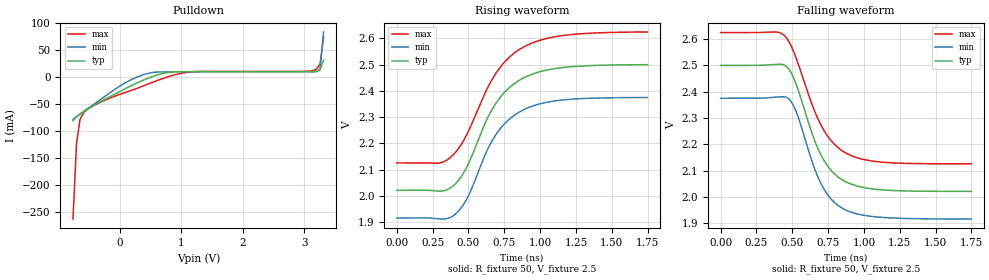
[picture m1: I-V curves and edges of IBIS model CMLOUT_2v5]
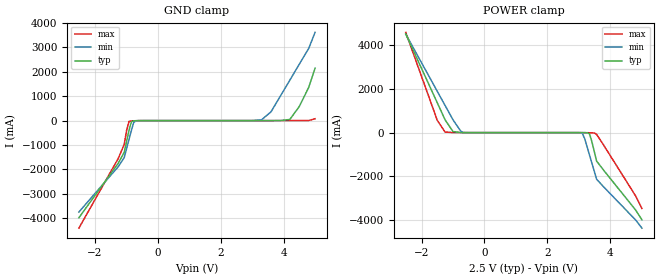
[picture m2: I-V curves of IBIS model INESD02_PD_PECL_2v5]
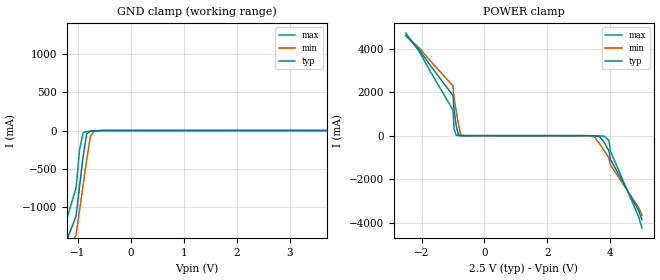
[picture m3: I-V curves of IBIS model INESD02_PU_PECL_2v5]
|   This file is an IBIS representation of the   |
|   Integrated Devices Technolog, Inc.   |
|   ICS845252I   |
|   FEMTOCLOCK CRYSTAL-TO-CML CLOCK GENERATOR   |
[IBIS Ver]   4.1
[File name]   845252i.ibs
[File Rev]   1
[Date]   9 Aug 2010
[Source]   Originated at Integrated Device Technology, Inc.
[Disclaimer]
IDT hereby grants the user of this IBIS model a non-exclusive,
nontransferable license to use this IBIS model under the following terms.
Before using this IBIS model, the user should read this license.
If the user does not accept these terms,  the IBIS model should be
returned to IDT within 30 days.
   The user is granted this license only to use the IBIS model and
is not granted rights to sell, load, rent, lease or license the IBIS
model in whole or in part, or in modified form to anyone other than
user. User may modify the IBIS model to suit its specific
applications but rights to derivative works and such modifications
shall belong to IDT.
   This IBIS model is provided on an "AS IS" basis and IDT makes
absolutely no warranty with respect to the information contained
herein. IDT DISCLAIMS AND CUSTOMER WAIVES ALL WARRANTIES, EXPRESS
OR IMPLIED, INCLUDING WARRANTIES OF MERCHANTABILITY OR FITNESS FOR
A PARTICULAR PURPOSE. The entire risk as to quality and performance
is with the Customer. ACCORDINGLY, IN NO EVENT SHALL THE COMPANY BE
LIABLE FOR ANY DAMAGES, WHETHER IN CONTRACT OR TORT,INCLUDING ANY
LOST PROFITS OR OTHER INCIDENTAL, CONSEQUENTIAL, EXEMPLARY, OR
PUNITIVE DAMAGES ARISING OUT OF THE USE OR APPLICATION OF THE IBIS
model provided in this package. Further, IDT reserves the right to
make changes without notice to any product herein to improve
reliability, function, or design. IDT does not convey any license
under patent rights or any other intellectual property rights,
including those of third parties.
   IDT is not obligated to provide maintenance or support
for the licensed IBIS model.
[Copyright]   Copyright 2010 by Integrated Device Technology, Inc.
[Component]   ICS845252KI
[Manufacturer] Integrated Device Technology, Inc.
[Package]
|LD QFN 32
|lead+wire  typ   min   max
R_pkg   72.4655m   58.886m   86.045m
L_pkg   1.47175nH   1.11650nH   1.77850n
C_pkg   0.07747pF   0.07444pF   0.08050p
[Pin]   signal_name   model_name  R_pin   L_pin   C_pin
1  nQ0   CMLOUT   86.045m   1.77850n  0.08050pF
2  Q0   CMLOUT   76.996m   1.55783n  0.07848pF
3  VDD   POWER   67.941m   1.33717n  0.07646pF
4  nOE   INESD02_PD_PECL   58.886m   1.11650n  0.07444pF
5  NC   NC   58.886m   1.11650n  0.07444pF
6  NC   NC   67.941m   1.33717n  0.07646pF
7  NC   NC   76.996m   1.55783n  0.07848pF
8  NC   NC   86.045m   1.77850n  0.08050pF
9  NC   NC   86.045m   1.77850n  0.08050pF
10 VDDA   POWER   76.996m   1.55783n  0.07848pF
11 nBYPASS  INESD02_PU_PECL   67.941m   1.33717n  0.07646pF
12 REF_CLK  INESD02_PD_PECL   58.886m   1.11650n  0.07444pF
13 GND   GND   58.886m   1.11650n  0.07444pF
14 XTAL_OUT NC   67.941m   1.33717n  0.07646pF
15 XTAL_IN  NC   76.996m   1.55783n  0.07848pF
16 NC   NC   86.045m   1.77850n  0.08050pF
17 NC   NC   86.045m   1.77850n  0.08050pF
18 VDD   POWER   76.996m   1.55783n  0.07848pF
19 NC   NC   67.941m   1.33717n  0.07646pF
20 FSEL0   INESD02_PD_PECL   58.886m   1.11650n  0.07444pF
21 FSEL1   INESD02_PD_PECL   58.886m   1.11650n  0.07444pF
22 REF_SEL  INESD02_PD_PECL   67.941m   1.33717n  0.07646pF
23 NC   NC   76.996m   1.55783n  0.07848pF
24 NC   NC   86.045m   1.77850n  0.08050pF
25 NC   NC   86.045m   1.77850n  0.08050pF
26 FBSEL   INESD02_PD_PECL   76.996m   1.55783n  0.07848pF
27 nQ1   CMLOUT   67.941m   1.33717n  0.07646pF
28 Q1   CMLOUT   58.886m   1.11650n  0.07444pF
29 GND   GND   58.886m   1.11650n  0.07444pF
30  NC   NC   67.941m   1.33717n  0.07646pF
31  NC   NC   76.996m   1.55783n  0.07848pF
32  NC   NC   86.045m   1.77850n  0.08050pF
[Diff Pin]  inv_pin  vdiff tdelay_typ tdelay_min  tdelay_max
2   1   NA   0   0   0
28   27   NA   0   0   0
[Model Selector] CMLOUT
CMLOUT_2v5  Buffer selection for 2v5
CMLOUT_3v3  Buffer selection for 3v3
[Model Selector] INESD02_PD_PECL
INESD02_PD_PECL_2v5  Buffer selection for 2v5
INESD02_PD_PECL_3v3  Buffer selection for 3v3
[Model Selector] INESD02_PU_PECL
INESD02_PU_PECL_2v5  Buffer selection for 2v5
INESD02_PU_PECL_3v3  Buffer selection for 3v3
| Models and submodels in the file (6): CMLOUT_2v5 (Open_drain), INESD02_PD_PECL_2v5 (Input), INESD02_PU_PECL_2v5 (Input), CMLOUT_3v3 (Open_drain), INESD02_PD_PECL_3v3 (Input), INESD02_PU_PECL_3v3 (Input)
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[Model] CMLOUT_2v5
Model_type   Open_drain
Polarity   Non-Inverting
|   typ   min   max
C_comp   2pF   1.5pF   2.5pF
Vmeas = 2.27V
Rref = 50
Cref = 0
Vref = 2.5V
|   typ   min   max
[Voltage range]   3.3V   3.135V   3.465V
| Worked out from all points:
|   slope of the pulldown table from 0 to 0.495 V, typ, clamps not added: 18.9 ohm
|   rising waveform, R_fixture 50, V_fixture 2.5: 20-80 % time 274ps typ, 261ps min, 298ps max; typ from 2.02 V to 2.5 V
|   falling waveform, R_fixture 50, V_fixture 2.5: 20-80 % time 205ps typ, 194ps min, 225ps max; typ from 2.5 V to 2.02 V
[Pulldown]
|Voltage   I (typ)   I (min)   I (max)
|Note, modeling breaks down at 250mA and above.  This is well beyond the functional   |
|operating range of the device.  Should this scenario occur, catastrophic failure and   |
|possible damage to the device and/or board is of higher concern than the I-V curve   |
|behavior.  The IBIS checker will flag currents in excess of 10A with warnings.  Lines   |
|with currents in excess of 0.35 A have been commented out.  The points still remain|
|available to the user if the user desires to use them.   |
|-2.20000e+00   -4.94553e+00   -5.82756e+00   -4.17575e+00
|-1.90000e+00   -3.86454e+00   -4.45984e+00   -3.35552e+00
|-1.60000e+00   -2.78212e+00   -3.09582e+00   -2.53344e+00
|-1.30000e+00   -1.70862e+00   -1.74462e+00   -1.71123e+00
|-1.00000e+00   -6.47434e-01   -3.95497e-01   -8.99844e-01
|-9.90000e-01   -6.12107e-01   -3.50581e-01   -8.73149e-01
|-9.32644e-01   -4.09577e-01   -1.27771e-01   -7.20243e-01
|-8.75287e-01   -2.07199e-01   -9.22212e-02   -5.67577e-01
|-8.17931e-01   -9.83237e-02   -8.44918e-02   -4.15088e-01
-760.6mV  -81.03mA   -78.71mA   -262.8mA
-703.2mV  -74.35mA   -73.45mA   -123.2mA
-645.9mV  -69.13mA   -68.57mA   -78.53mA
-531.1mV  -60.14mA   -59.39mA   -60.59mA
99.77mV   -21.24mA   -10.5mA    -28.49mA
501.3mV   -828.2uA   7.403mA    -11.48mA
788mV     8.086mA    9.146mA    190.5uA
1.132V    9.554mA    9.171mA    8.802mA
2.968V    9.574mA    9.177mA    10.07mA
3.197V    10.3mA     9.537mA    14.09mA
3.254V    12.77mA    13.73mA    24.14mA
3.312V    31.13mA    82.92mA    72.69mA
| 3.36908e+00   1.94882e-01   6.90130e-01   3.21665e-01
| 3.42644e+00   7.71281e-01   1.44758e+00   7.66427e-01
| 3.48379e+00   1.36443e+00   2.20531e+00   1.21136e+00
| 3.54115e+00   1.95779e+00   2.96327e+00   1.65643e+00
| 3.59851e+00   2.55133e+00   3.72144e+00   2.10164e+00
| 3.65586e+00   3.14502e+00   4.47980e+00   2.54696e+00
| 3.71322e+00   3.73886e+00   5.23831e+00   2.99240e+00
| 3.77057e+00   4.33282e+00   5.99697e+00   3.43793e+00
| 3.82793e+00   4.92690e+00   6.75576e+00   3.88354e+00
| 3.88529e+00   5.52108e+00   7.51466e+00   4.32924e+00
| 3.94264e+00   6.11535e+00   8.27367e+00   4.77501e+00
| 4.00000e+00   6.70970e+00   9.03277e+00   5.22086e+00
| 4.01000e+00   6.81334e+00   9.16512e+00   5.29859e+00
| 4.20800e+00   8.86569e+00   1.17862e+01   6.83817e+00
| 4.40600e+00   1.09187e+01   1.44080e+01   8.37830e+00
| 4.60400e+00   1.29722e+01   1.70303e+01   9.91887e+00
| 4.80200e+00   1.50260e+01   1.96529e+01   1.14598e+01
| 5.00000e+00   1.70800e+01   2.22758e+01   1.30010e+01
[Ramp]
|   typ   min   max
dV/dt_r   0.288/0.274n   0.277/0.262n   0.299/0.298n
dV/dt_f   0.29/0.205n   0.279/0.195n   0.301/0.225n
R_load =   50.0000
[Rising Waveform]
R_fixture = 50
V_fixture = 2.5
V_fixture_min = 2.375
V_fixture_max = 2.625
C_fixture = 0.0p
| Time   typ   min   max
0s        2.022V     1.916V     2.126V
297.8ps   2.019V     1.913V     2.126V
408.2ps   2.046V     1.931V     2.166V
494ps     2.116V     1.995V     2.24V
620.1ps   2.282V     2.162V     2.397V
688.4ps   2.35V      2.231V     2.464V
781.3ps   2.41V      2.29V      2.526V
895.1ps   2.452V     2.331V     2.57V
1.188ns   2.49V      2.367V     2.612V
1.748ns   2.5V       2.375V     2.624V
[Falling Waveform]
R_fixture = 50
V_fixture = 2.5
V_fixture_min = 2.375
V_fixture_max = 2.625
C_fixture = 0.0p
| Time   typ   min   max
0s        2.5V       2.375V     2.625V
395.9ps   2.504V     2.38V      2.627V
476.5ps   2.486V     2.372V     2.59V
530.8ps   2.423V     2.319V     2.522V
637.6ps   2.241V     2.135V     2.352V
700.7ps   2.159V     2.05V      2.272V
779.5ps   2.095V     1.987V     2.208V
881.1ps   2.055V     1.948V     2.165V
1.139ns   2.026V     1.921V     2.131V
1.748ns   2.021V     1.916V     2.125V
[Model] INESD02_PD_PECL_2v5
Model_type   Input
Polarity   Non-Inverting
Vinl = 0.8V
Vinh = 2.0V
|   typ   min   max
C_comp   2pF   1.5pF   2.5pF
|   typ   min   max
[Voltage range]  2.5V   2.375V   2.625V
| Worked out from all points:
|   GND clamp passes 1 mA (typ) near -0.59 V on its own axis
|   POWER clamp passes 1 mA (typ) near -0.69 V on its own axis
[GND_clamp]
|Voltage   I(typ)   I(min)   I(max)
-2.5V     -3.983A    -3.749A    -4.408A
-1.25V    -1.747A    -1.889A    -1.551A
-1.061V   -1.3A      -1.517A    -979.1mA
-909.1mV  -407.1mA   -774.3mA   -35.24mA
-833.3mV  -48.47mA   -403.4mA   -14.47mA
-757.6mV  -7.272mA   -70.21mA   -9.677mA
-681.8mV  -2.863mA   -7.067mA   -5.73mA
3.3V      167.2uA    32.81mA    49.66uA
3.6V      586.4uA    357.8mA    70.1uA
4.2V      47.81mA    1.661A     649.6uA
4.8V      1.366A     2.965A     5.596mA
5V        2.15A      3.618A     75.79mA
[POWER_clamp]
|Voltage   I(typ)   I(min)   I(max)
-2.5V     4.503A     4.499A     4.579A
-1.5V     1.366A     1.889A     566.5mA
-1.25V    582.4mA    1.237A     24.21mA
-1V       47.81mA    585.7mA    3.595mA
-681.8mV  586.4uA    6.896mA    416.8uA
3.03V     -323.1uA   -3.378mA   -47.98uA
3.106V    -1.127mA   -30.71mA   -286.5uA
3.182V    -2.863mA   -273.7mA   -1.276mA
3.333V    -48.47mA   -1.016A    -7.036mA
3.561V    -1.3A      -2.13A     -81.94mA
4.8V      -3.536A    -3.991A    -2.894A
5V        -3.983A    -4.363A    -3.465A
[Model] INESD02_PU_PECL_2v5
Model_type   Input
Polarity   Non-Inverting
Vinl = .8V
Vinh =  2V
|   typ   min   max
C_comp   2pF   1.5pF   2.5pF
|   typ   min   max
[Voltage range]  2.5V   2.375V   2.625V
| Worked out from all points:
|   GND clamp passes 1 mA (typ) near -0.59 V on its own axis
|   POWER clamp passes 1 mA (typ) near -0.70 V on its own axis
[GND_clamp]
|Voltage   I(typ)   I(min)   I(max)
-2.5V     -3.894A    -3.674A    -4.294A
-1.25V    -1.521A    -1.7A      -1.261A
-1.031V   -1.125A    -1.372A    -755.3mA
-896.9mV  -335.4mA   -714.7mA   -27.06mA
-695.9mV  -3.401mA   -10.7mA    -6.467mA
3.995V    711.6uA    10.32mA    481.3uA
4.062V    4.029mA    88.04mA    1.401mA
4.129V    40.44mA    547.3mA    3.341mA
4.196V    445.8mA    1.124A     14.79mA
4.263V    1.139A     1.7A       275.9mA
4.5V      1.832A     2.277A     1.163A
5V        3.219A     3.431A     2.937A
[POWER_clamp]
|Voltage   I(typ)   I(min)   I(max)
-2.5V     4.617A     4.594A     4.726A
-1V       1.842A     2.286A     1.176A
-963.9mV  1.149A     1.709A     289.6mA
-896.9mV  456.4mA    1.132A     15.33mA
-829.9mV  42.02mA    556.1mA    3.389mA
-762.9mV  4.159mA    91.01mA    1.421mA
-695.9mV  727.9uA    10.67mA    490.4uA
3.35V     -3.204mA   -9.193mA   -6.2mA
3.8V      -305mA     -689.5mA   -24.7mA
3.95V     -699.9mA   -1.018A    -211mA
4V        -1.095A    -1.346A    -716.4mA
5V        -3.863A    -3.649A    -4.255A
